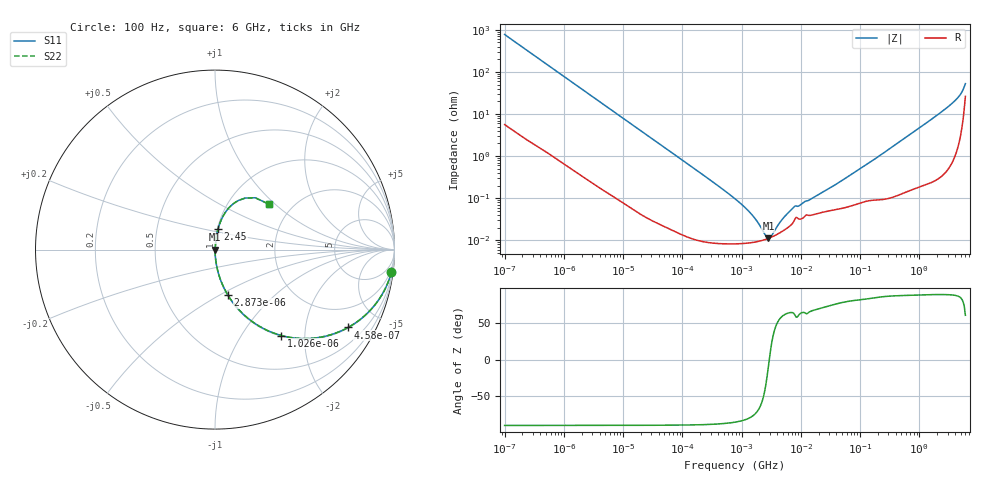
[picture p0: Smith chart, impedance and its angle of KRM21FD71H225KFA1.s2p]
!Murata Part Number: KRM21FD71H225KFA1
!These Parameters are Measured in Series Mode Connection
!Data Generated on Jan 08, 2026
!  o--ll--o
!Port1  Port2
!  o------o
!Operation Temp=25[degC], DC Bias Voltage=0[V]
!Freq. Start=100[Hz] Stop=6[GHz] 401[Steps]
# Hz S RI R 50
!Freq.(Hz) S11(Real) S11(Imag) S21(Real) S21(Imag) S12(Real) S12(Imag) S22(Real) S22(Imag)
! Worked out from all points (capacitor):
!   401 points, 100 Hz to 6 GHz, reference 50 ohm
!   read as one part in series: C = 2.05 uF near 109 Hz
!   lowest |Z| = 11.3 mohm at 2.838 MHz (marker M1)
!   series resonance near 2.936 MHz, so ESL is about 1.4 nH
!   S11 on the Smith chart (normalised r, x): 100 Hz: 1, -16; 458 Hz: 1.03, -3.41; 1.026 kHz: 1.01, -1.53; 2.873 kHz: 1.00, -0.55; 2.45 GHz: 1.01, +0.23; 6 GHz: 1.52, +0.91
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100  0.9827 -0.1267  0.0173 0.1267  0.0173 0.1267  0.9827 -0.1267
245  0.9082 -0.285  0.0918 0.285  0.0918 0.285  0.9082 -0.285
458  0.7421 -0.4335  0.2579 0.4335  0.2579 0.4335  0.7421 -0.4335
686  0.5651 -0.4916  0.4349 0.4916  0.4349 0.4916  0.5651 -0.4916
1026  0.3698 -0.4786  0.6302 0.4786  0.6302 0.4786  0.3698 -0.4786
2008  0.1353 -0.3377  0.8647 0.3377  0.8647 0.3377  0.1353 -0.3377
2873  0.0719 -0.2541  0.9281 0.2541  0.9281 0.2541  0.0719 -0.2541
8801  0.00891 -0.0893  0.9911 0.0893  0.9911 0.0893  0.00891 -0.0893
40335  0.000637 -0.0198  0.9994 0.0198  0.9994 0.0198  0.000637 -0.0198
774597  8.34e-05 -0.000968  0.9999 0.000968  0.9999 0.000968  8.34e-05 -0.000968
1516199  8.89e-05 -0.000387  0.9999 0.000387  0.9999 0.000387  8.89e-05 -0.000387
2481164  0.000104 -9.1e-05  0.9999 9.1e-05  0.9999 9.1e-05  0.000104 -9.1e-05
2837864  0.000111 -1.81e-05  0.9999 1.81e-05  0.9999 1.81e-05  0.000111 -1.81e-05
3245845  0.00012 5.34e-05  0.9999 -5.34e-05  0.9999 -5.34e-05  0.00012 5.34e-05
4643984  0.000157 0.000245  0.9998 -0.000245  0.9998 -0.000245  0.000157 0.000245
7266822  0.000255 0.000516  0.9997 -0.000516  0.9997 -0.000516  0.000255 0.000516
1.555665e7  0.000401 0.000913  0.9996 -0.000913  0.9996 -0.000913  0.000401 0.000913
4.556224e7  0.000566 0.00238  0.9994 -0.00238  0.9994 -0.00238  0.000566 0.00238
3.124326e8  0.00122 0.0148  0.9988 -0.0148  0.9988 -0.0148  0.00122 0.0148
2.450438e9  0.0167 0.1141  0.9833 -0.1141  0.9833 -0.1141  0.0167 0.1141
4.586474e9  0.0756 0.2306  0.9244 -0.2306  0.9244 -0.2306  0.0756 0.2306
6e9  0.2993 0.2534  0.7007 -0.2534  0.7007 -0.2534  0.2993 0.2534
